FUNCTION "TD_17PRESS" : VOID
TITLE =BLOCK TD_17 PRESS
AUTHOR : Esposito
FAMILY : EGAL_srl
NAME : TD_17PRE
VERSION : 0.1

BEGIN
NETWORK
TITLE =CAMBIO PAGINA
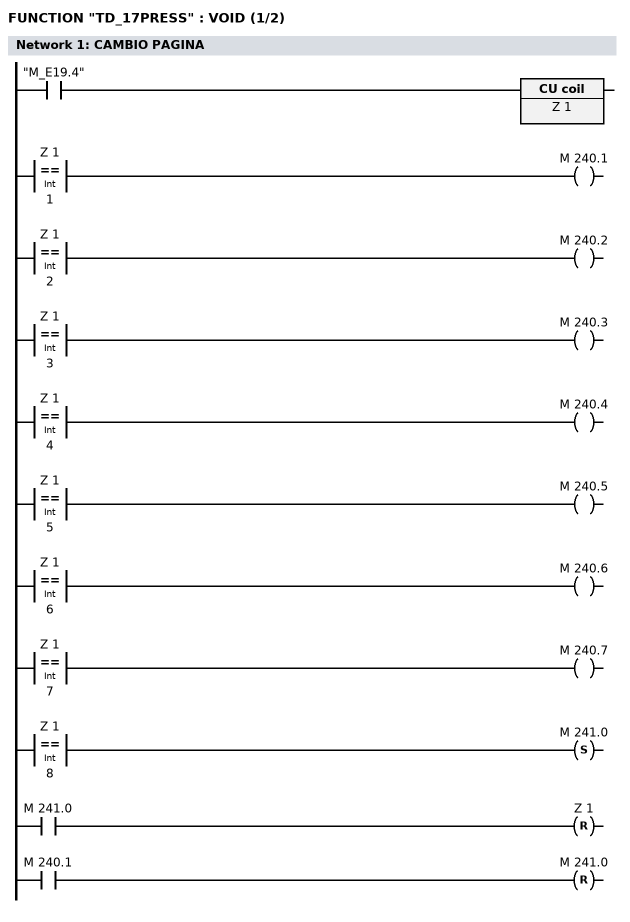
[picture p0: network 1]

      U     "M_E19.4";
      ZV    Z      1;

      L     Z      1;
      L     1;
      ==I   ;
      =     M    240.1;

      L     Z      1;
      L     2;
      ==I   ;
      =     M    240.2;

      L     Z      1;
      L     3;
      ==I   ;
      =     M    240.3;

      L     Z      1;
      L     4;
      ==I   ;
      =     M    240.4;

      L     Z      1;
      L     5;
      ==I   ;
      =     M    240.5;

      L     Z      1;
      L     6;
      ==I   ;
      =     M    240.6;

      L     Z      1;
      L     7;
      ==I   ;
      =     M    240.7;

      L     Z      1;
      L     8;
      ==I   ;
      S     M    241.0;

      U     M    241.0;
      R     Z      1;

      U     M    240.1;
      R     M    241.0;

NETWORK
TITLE =START PAGES TD_17 PRESS
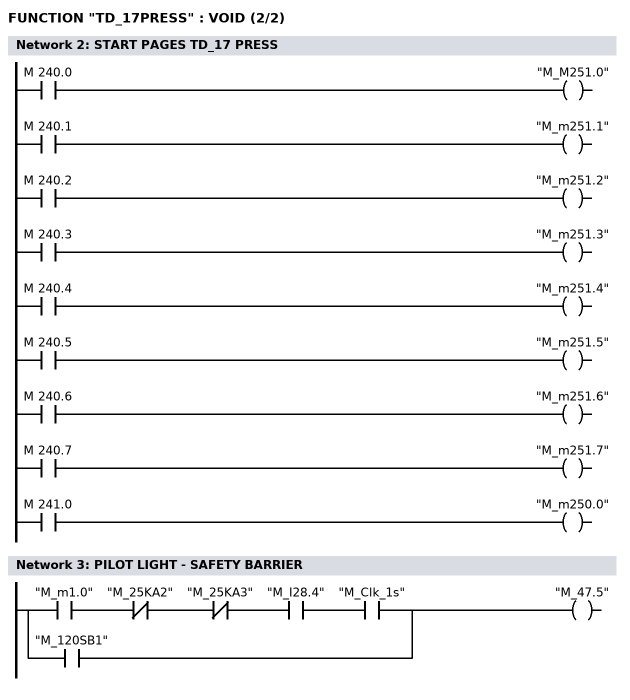
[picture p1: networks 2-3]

      U     M    240.0;
      =     "M_M251.0";

      U     M    240.1;
      =     "M_m251.1";

      U     M    240.2;
      =     "M_m251.2";

      U     M    240.3;
      =     "M_m251.3";

      U     M    240.4;
      =     "M_m251.4";

      U     M    240.5;
      =     "M_m251.5";

      U     M    240.6;
      =     "M_m251.6";

      U     M    240.7;
      =     "M_m251.7";

      U     M    241.0;
      =     "M_m250.0";
NETWORK
TITLE =PILOT LIGHT - SAFETY BARRIER

      U     "M_m1.0";
      UN    "M_25KA2";
      UN    "M_25KA3";
      U     "M_I28.4";
      U     "M_Clk_1s";
      O     "M_120SB1";
      =     "M_47.5";
END_FUNCTION

